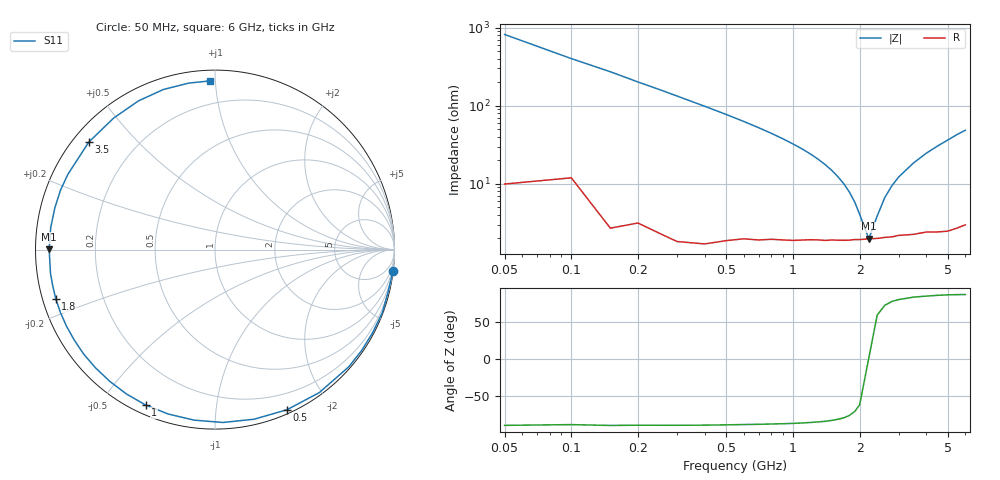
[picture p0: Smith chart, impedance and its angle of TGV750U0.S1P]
! SIEMENS Discrete & RF Semiconductors
! BAT64
! Si Schottky Diode in SOT23
! VR = 0.75 V
! S-Parameters:  February  1997
# GHz  S  MA  R  50
!  f  S11
! GHz  MAG  ANG
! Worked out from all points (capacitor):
!   34 points, 50 MHz to 6 GHz, reference 50 ohm
!   read as one part to ground: C = 3.89 pF near 50 MHz
!   lowest |Z| = 1.98 ohm at 2.2 GHz (marker M1)
!   series resonance near 2.198 GHz, so ESL is about 1.3 nH
!   S11 on the Smith chart (normalised r, x): 50 MHz: 0, -16; 500 MHz: 0.04, -1.55; 1 GHz: 0.04, -0.65; 1.8 GHz: 0.04, -0.15; 3.5 GHz: 0.05, +0.37; 6 GHz: 0.06, +0.97
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0.05  0.9985 -7.0
0.15  0.9965 -20.8
0.2  0.9927 -27.9
0.3  0.991 -41.2
0.4  0.9861 -53.9
0.5  0.9781 -65.8
0.6  0.9698 -77.0
0.7  0.9642 -87.4
0.8  0.9572 -97.0
0.9  0.9525 -105.9
1  0.9483 -114.1
1.1  0.9436 -121.6
1.2  0.9394 -128.7
1.3  0.9366 -135.3
1.4  0.935 -141.5
1.6  0.9309 -152.8
1.8  0.9284 -162.8
2  0.926 -171.8
2.2  0.924 179.9
2.4  0.9235 172.4
2.6  0.9221 165.4
3  0.9207 152.9
3.5  0.9237 139.6
4  0.9252 127.6
4.5  0.9318 117.2
5  0.9373 107.9
5.5  0.9392 99.0
6  0.9404 91.7
